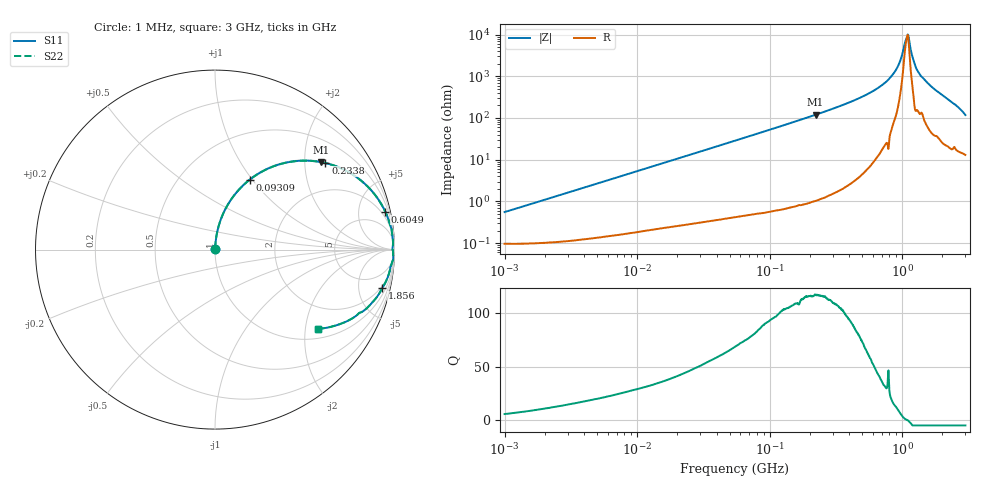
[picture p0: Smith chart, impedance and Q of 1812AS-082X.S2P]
!s-Parameter Generated by FASTRON Sdn. Bhd.
!FASTRON P/N : 1812AS-082X
!Keysight Technologies,E4991B,MY54100416,A.01.15
!Date created: Fri Oct 13 14:31:13 2023
!Version  : Rev00 Fri Oct 13 14:31:13 2023
!Data & Calibration Information:
!Freq	S11	S21	S12	S22
!PortZ  Port1:50+j0  Port2:50+j0
!When reading, reference impedance value at option line is always used.
! Remarks : This data is being provided solely for informational purposes.
# Hz S dB R 50
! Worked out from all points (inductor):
!   1601 points, 1 MHz to 3 GHz, reference 50 ohm
!   read as one part in series: L = 86.9 nH near 1.041 MHz
!   highest Q = 116 at 222.4 MHz (marker M1), where L = 85.8 nH
!   self-resonance near 1.092 GHz
!   S11 on the Smith chart (normalised r, x): 1 MHz: 1.00, +0.01; 93.09 MHz: 1.01, +0.97; 233.8 MHz: 1.02, +2.53; 604.9 MHz: 1.17, +8.92; 1.856 GHz: 1.69, -8.54; 3 GHz: 1.26, -2.35
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1000000  -45.12 79.7  -0.01 -0.3  -0.01 -0.3  -45.12 79.7
3804036  -33.76 85.5  -0.01 -1.2  -0.01 -1.2  -33.76 85.5
1.447069e7  -22.38 84.0  -0.04 -4.4  -0.04 -4.4  -22.38 84.0
5.477226e7  -11.25 73.3  -0.38 -15.9  -0.38 -15.9  -11.25 73.3
9.309362e7  -7.21 63.5  -0.96 -25.8  -0.96 -25.8  -7.21 63.5
2.083556e8  -2.59 41.6  -3.56 -47.9  -3.56 -47.9  -2.59 41.6
2.223601e8  -2.33 39.6  -3.91 -49.9  -3.91 -49.9  -2.33 39.6
2.3377e8  -2.14 38.1  -4.19 -51.4  -4.19 -51.4  -2.14 38.1
3.973271e8  -0.75 22.9  -8.20 -66.5  -8.20 -66.5  -0.75 22.9
6.049187e8  -0.25 12.6  -13.24 -76.3  -13.24 -76.3  -0.25 12.6
7.925923e8  -0.08 6.6  -18.78 -81.9  -18.78 -81.9  -0.08 6.6
9.349007e8  -0.06 3.1  -25.28 -80.6  -25.28 -80.6  -0.06 3.1
9.828732e8  -0.07 2.0  -28.89 -76.9  -28.89 -76.9  -0.07 2.0
1.064802e9  -0.10 0.4  -37.37 -33.7  -37.37 -33.7  -0.10 0.4
1.091779e9  -0.09 0.1  -39.51 -6.6  -39.51 -6.6  -0.09 0.1
1.130699e9  -0.07 -0.6  -37.18 54.2  -37.18 54.2  -0.07 -0.6
1.231095e9  -0.05 -2.6  -26.81 81.3  -26.81 81.3  -0.05 -2.6
1.320433e9  -0.10 -4.4  -22.28 79.2  -22.28 79.2  -0.10 -4.4
1.54974e9  -0.19 -8.0  -17.12 77.0  -17.12 77.0  -0.19 -8.0
1.855641e9  -0.38 -12.9  -13.02 72.5  -13.02 72.5  -0.38 -12.9
2.468121e9  -1.13 -23.7  -7.88 61.0  -7.88 61.0  -1.13 -23.7
3e9  -2.80 -37.6  -4.24 46.1  -4.24 46.1  -2.80 -37.6
